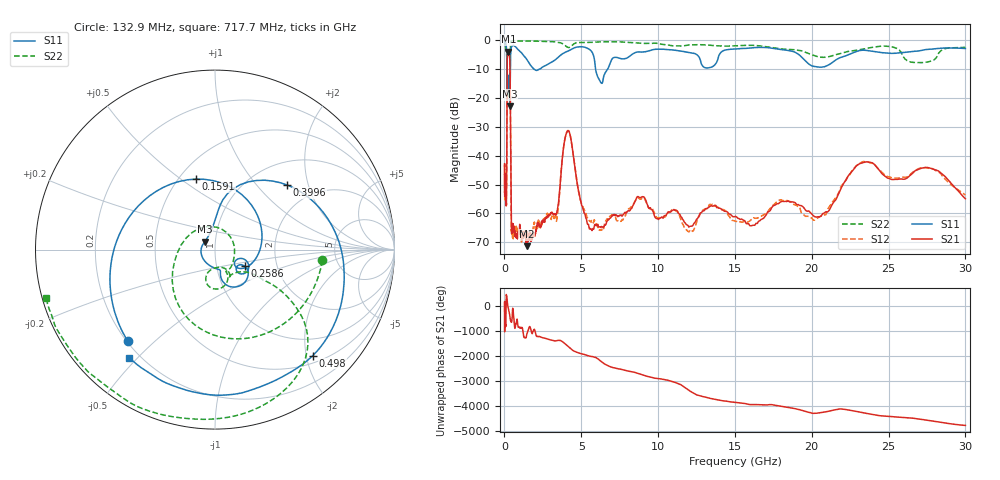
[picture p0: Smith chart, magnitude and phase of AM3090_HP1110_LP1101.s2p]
! Date/Time: Thu, Feb 28, 2019 2:09 PM
! Network Analyzer: Agilent Technologies E8364B Rev: A.07.50.67
! Sweep from 0.010 to 30.000 GHz, 1601 Points, Sweep Type: LOG
! Power Supply: 5.023 V, 0.002 A
# Hz S DB R 50
!freq MagS11 AngS11 MagS21 AngS21 MagS12 AngS12 MagS22 AngS22
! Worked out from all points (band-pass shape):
!   1601 points, 10 MHz to 30 GHz, reference 50 ohm
!   highest |S21| = -3.95 dB at 253.4 MHz (marker M1); lowest = -71.3 dB at 1.446 GHz (marker M2)
!   |S21| within 3 dB of the highest: 177.9 MHz to 348.8 MHz (170.9 MHz wide, 64.9 % of centre)
!   lowest |S11| = -22.9 dB at 354.4 MHz (marker M3), VSWR 1.15, Z = 44.5 + j3.96 ohm
!   |S11| at or under -10 dB: 166 MHz to 383.9 MHz (217.9 MHz wide, 79.2 % of centre); 1.903 GHz to 2.268 GHz (364.5 MHz wide, 17.5 % of centre); 5.93 GHz to 6.719 GHz (788.7 MHz wide, 12.5 % of centre)
!   |S22| runs from -20.0 to -0.1 dB; largest |S21 - S12| = 0.013
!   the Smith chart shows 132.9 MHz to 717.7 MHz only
!   S11 on the Smith chart (normalised r, x): 132.9 MHz: 0.20, -0.41; 159.1 MHz: 0.61, +0.57; 258.6 MHz: 1.37, -0.26; 399.6 MHz: 1.46, +1.48; 498 MHz: 0.64, -2.13; 717.7 MHz: 0.16, -0.47
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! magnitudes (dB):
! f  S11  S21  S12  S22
! 10 MHz  -0.3  -43.6  -46.4  -0.7
! 38.04 MHz  -0.3  -49.6  -52.1  -1.4
! 132.9 MHz  -3.0  -54.0  -52.6  -4.4
! 144.7 MHz  -4.5  -47.8  -48.3  -5.1
! 159.1 MHz  -7.8  -23.0  -23.1  -10.6
! 179.4 MHz  -13.8  -6.6  -6.6  -17.4
! 253.4 MHz  -15.4  -4.0  -3.9  -19.5
! 258.6 MHz  -14.5  -4.0  -3.9  -20.0
! 354.4 MHz  -22.9  -7.8  -7.7  -9.5
! 399.6 MHz  -5.4  -34.7  -34.7  -1.2
! 441.7 MHz  -2.7  -63.2  -62.9  -0.5
! 498 MHz  -1.9  -66.8  -66.4  -0.2
! 550.5 MHz  -1.9  -63.6  -67.9  -0.2
! 717.7 MHz  -2.3  -67.2  -66.3  -0.2
! 1.446 GHz  -6.7  -71.3  -67.3  -0.3
! 2.084 GHz  -10.5  -65.3  -65.6  -0.4
! 3.368 GHz  -6.5  -60.3  -62.6  -0.7
! 4.115 GHz  -3.8  -31.4  -31.3  -2.5
! 5.556 GHz  -3.3  -65.2  -62.7  -0.8
! 7.926 GHz  -6.3  -59.8  -59.5  -0.8
! 23.48 GHz  -3.5  -42.2  -42.1  -3.0
! 30 GHz  -2.9  -54.9  -53.6  -2.5
